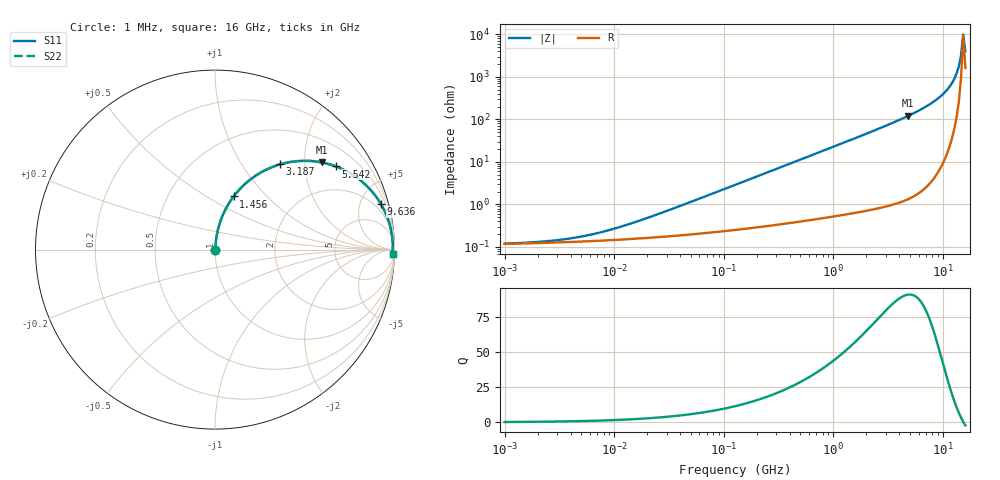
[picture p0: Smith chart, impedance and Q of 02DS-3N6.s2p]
# MHz S MA R 50
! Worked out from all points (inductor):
!   211 points, 1 MHz to 16 GHz, reference 50 ohm
!   read as one part in series: L = 3.6 nH near 22.98 MHz
!   highest Q = 90.3 at 4.826 GHz (marker M1), where L = 3.99 nH
!   self-resonance near 15.28 GHz
!   S11 on the Smith chart (normalised r, x): 1 MHz: 1.00, +0.00; 1.456 GHz: 1.01, +0.66; 3.187 GHz: 1.02, +1.51; 5.542 GHz: 1.03, +2.88; 9.636 GHz: 1.16, +7.18; 16 GHz: 33, -72
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1  0.0012 10.8  0.9988 -0.0  0.9988 -0.0  0.0012 10.8
2.51416  0.001377 24.3  0.9987 -0.0  0.9987 -0.0  0.001377 24.3
5.25662  0.001795 41.3  0.9987 -0.1  0.9987 -0.1  0.001795 41.3
10.4954  0.002789 58.1  0.9985 -0.1  0.9985 -0.1  0.002789 58.1
26.3872  0.0062 73.6  0.9983 -0.3  0.9983 -0.3  0.0062 73.6
132.458  0.02998 83.4  0.997 -1.7  0.997 -1.7  0.02998 83.4
333.021  0.07497 83.1  0.9938 -4.3  0.9938 -4.3  0.07497 83.1
664.915  0.1484 79.8  0.9846 -8.5  0.9846 -8.5  0.1484 79.8
1455.79  0.3137 70.7  0.9438 -18.3  0.9438 -18.3  0.3137 70.7
2204.33  0.4511 62.4  0.8859 -26.8  0.8859 -26.8  0.4511 62.4
3187.38  0.5982 52.6  0.794 -36.7  0.794 -36.7  0.5982 52.6
4826.25  0.767 39.3  0.6332 -50.1  0.6332 -50.1  0.767 39.3
5542.03  0.8173 34.5  0.5671 -54.8  0.5671 -54.8  0.8173 34.5
7652.55  0.9126 23.4  0.3964 -65.8  0.3964 -65.8  0.9126 23.4
9636.16  0.958 15.5  0.2667 -73.3  0.2667 -73.3  0.958 15.5
11587.3  0.9803 9.3  0.1615 -78.4  0.1615 -78.4  0.9803 9.3
12706.4  0.9867 6.2  0.1089 -79.9  0.1089 -79.9  0.9867 6.2
13305.8  0.9888 4.7  0.08262 -79.9  0.08262 -79.9  0.9888 4.7
13933.5  0.9902 3.2  0.05653 -78.4  0.05653 -78.4  0.9902 3.2
14590.9  0.9907 1.7  0.03091 -71.7  0.03091 -71.7  0.9907 1.7
15279.2  0.9906 0.2  0.01002 -19.4  0.01002 -19.4  0.9906 0.2
16000  0.9896 -1.3  0.02501 64.8  0.02501 64.8  0.9896 -1.3
